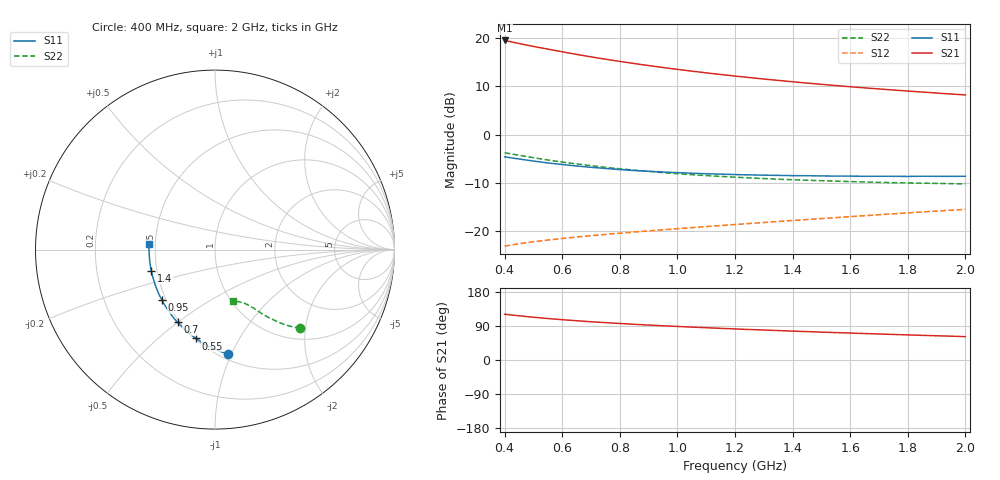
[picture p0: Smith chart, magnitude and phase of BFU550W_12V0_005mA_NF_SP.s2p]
! Filename:  P:\Prog\Test\Noise\ATS_data\Testdata_Net\06 Compressed Noise after Statistics\BFU550W_APM2013_11_D05_12p0V_005mA_NF_CM01_D.sf
! Date/Time: Tue 26/Mar/2013 16:25:25
! BFU550W_APM2013_11_D05_12p0V_1to35mA_NF_CM01_Bias4_R.sf
! Noise Parameter Data File
! BFU550W_APM2013_11_D05_12p0V_1to35mA_NF_CM01
! Date/time: Mon Mar 25 15:58:35 2013
! VAR V_out= 12.001000
! VAR I_out= 5.000000
! VAR V_in= 0.795400
! VAR I_in= 0.041305
! Device data file deembeded for feedlines and parallel
! Original file: \06 Compressed Noise after Statistics\BFU550W_APM2013_11_D05_12p0V_005mA_NF_CM01_R.sf
! Feed-files: PR019V01_070313_Feed1.s2p, PR019V01_070313_Feed2.s2p
! Parallel-file: PR019V01_070313_Par.s2p
# MHz S MA R 50
!  Freq-MHz  S11-mag  S11-arg  S21-mag  S21-arg  S12-mag  S12-arg  S22-mag  S22-arg
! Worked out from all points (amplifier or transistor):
!   37 points, 400 MHz to 2 GHz, reference 50 ohm
!   highest |S21| = 19.6 dB at 400 MHz (marker M1)
!   |S21| within 3 dB of that: start of sweep to 659.8 MHz
!   unconditionally stable (mu >= 1): 1.774 GHz to end of sweep
!   at 500 MHz: K = 0.51, MSG = 20.3 dB, |S12| = -22.3 dB
!   at 1.1 GHz: K = 0.86, MSG = 16.0 dB, |S12| = -19.1 dB
!   at 2 GHz: K = 1.02, MAG = 11.1 dB, |S12| = -15.6 dB
!   lowest NFmin = 0.60 dB at 420 MHz
!   S11 on the Smith chart (normalised r, x): 400 MHz: 0.55, -0.97; 550 MHz: 0.51, -0.68; 700 MHz: 0.49, -0.50; 950 MHz: 0.47, -0.32; 1.4 GHz: 0.47, -0.13; 2 GHz: 0.46, +0.03
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400  0.5867 -82.8  9.501 120.8  0.06906 54.6  0.646 -42.6
420  0.5738 -85.7  9.227 119.1  0.07082 54.0  0.6309 -43.6
440  0.5622 -88.5  8.968 117.4  0.07241 53.4  0.6158 -44.5
460  0.5514 -91.1  8.709 115.9  0.07391 53.0  0.6013 -45.3
500  0.53 -96.2  8.237 112.9  0.07674 52.1  0.5742 -46.9
550  0.5063 -102.0  7.722 109.4  0.07994 51.5  0.5434 -48.5
600  0.4878 -107.5  7.243 106.3  0.08305 51.0  0.5167 -49.8
650  0.4706 -112.4  6.803 103.6  0.08597 50.8  0.4948 -51.0
700  0.4558 -117.2  6.419 101.0  0.08877 50.6  0.4739 -52.1
750  0.4441 -121.5  6.067 98.6  0.0915 50.7  0.456 -53.0
800  0.4321 -125.7  5.753 96.3  0.09422 50.8  0.4403 -53.9
850  0.4226 -129.7  5.468 94.2  0.09689 50.9  0.4256 -54.6
950  0.4073 -136.7  4.973 90.3  0.1022 51.4  0.4016 -56.0
1050  0.3961 -143.2  4.558 86.8  0.1076 52.1  0.3821 -57.3
1100  0.3911 -146.1  4.376 85.2  0.1104 52.4  0.3741 -57.9
1200  0.3836 -151.8  4.054 82.0  0.116 53.0  0.3602 -59.2
1300  0.3779 -157.0  3.775 79.1  0.1217 53.6  0.3483 -60.3
1400  0.3736 -161.8  3.535 76.2  0.1277 54.2  0.3389 -61.5
1500  0.3709 -166.2  3.324 73.6  0.1338 54.8  0.3311 -63.0
1600  0.3694 -170.4  3.138 71.1  0.14 55.3  0.3242 -64.3
1750  0.3678 -176.0  2.901 67.4  0.1498 56.0  0.3156 -66.3
2000  0.3684 175.3  2.579 61.7  0.1668 56.6  0.3068 -70.4
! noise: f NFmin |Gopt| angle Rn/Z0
400  0.601  0.1573  48.63  0.1021
460  0.6378  0.1685  52.83  0.0997
600  0.6576  0.1716  55.9  0.1096
800  0.7137  0.1902  80.38  0.0943
1000  0.7342  0.2089  93.87  0.093
1200  0.7889  0.2333  109.2  0.0861
1400  0.8328  0.2471  122.6  0.0755
1600  0.8116  0.2609  137.2  0.0764
1800  0.8666  0.2776  150.8  0.0714
2000  0.9527  0.2995  165  0.0648
